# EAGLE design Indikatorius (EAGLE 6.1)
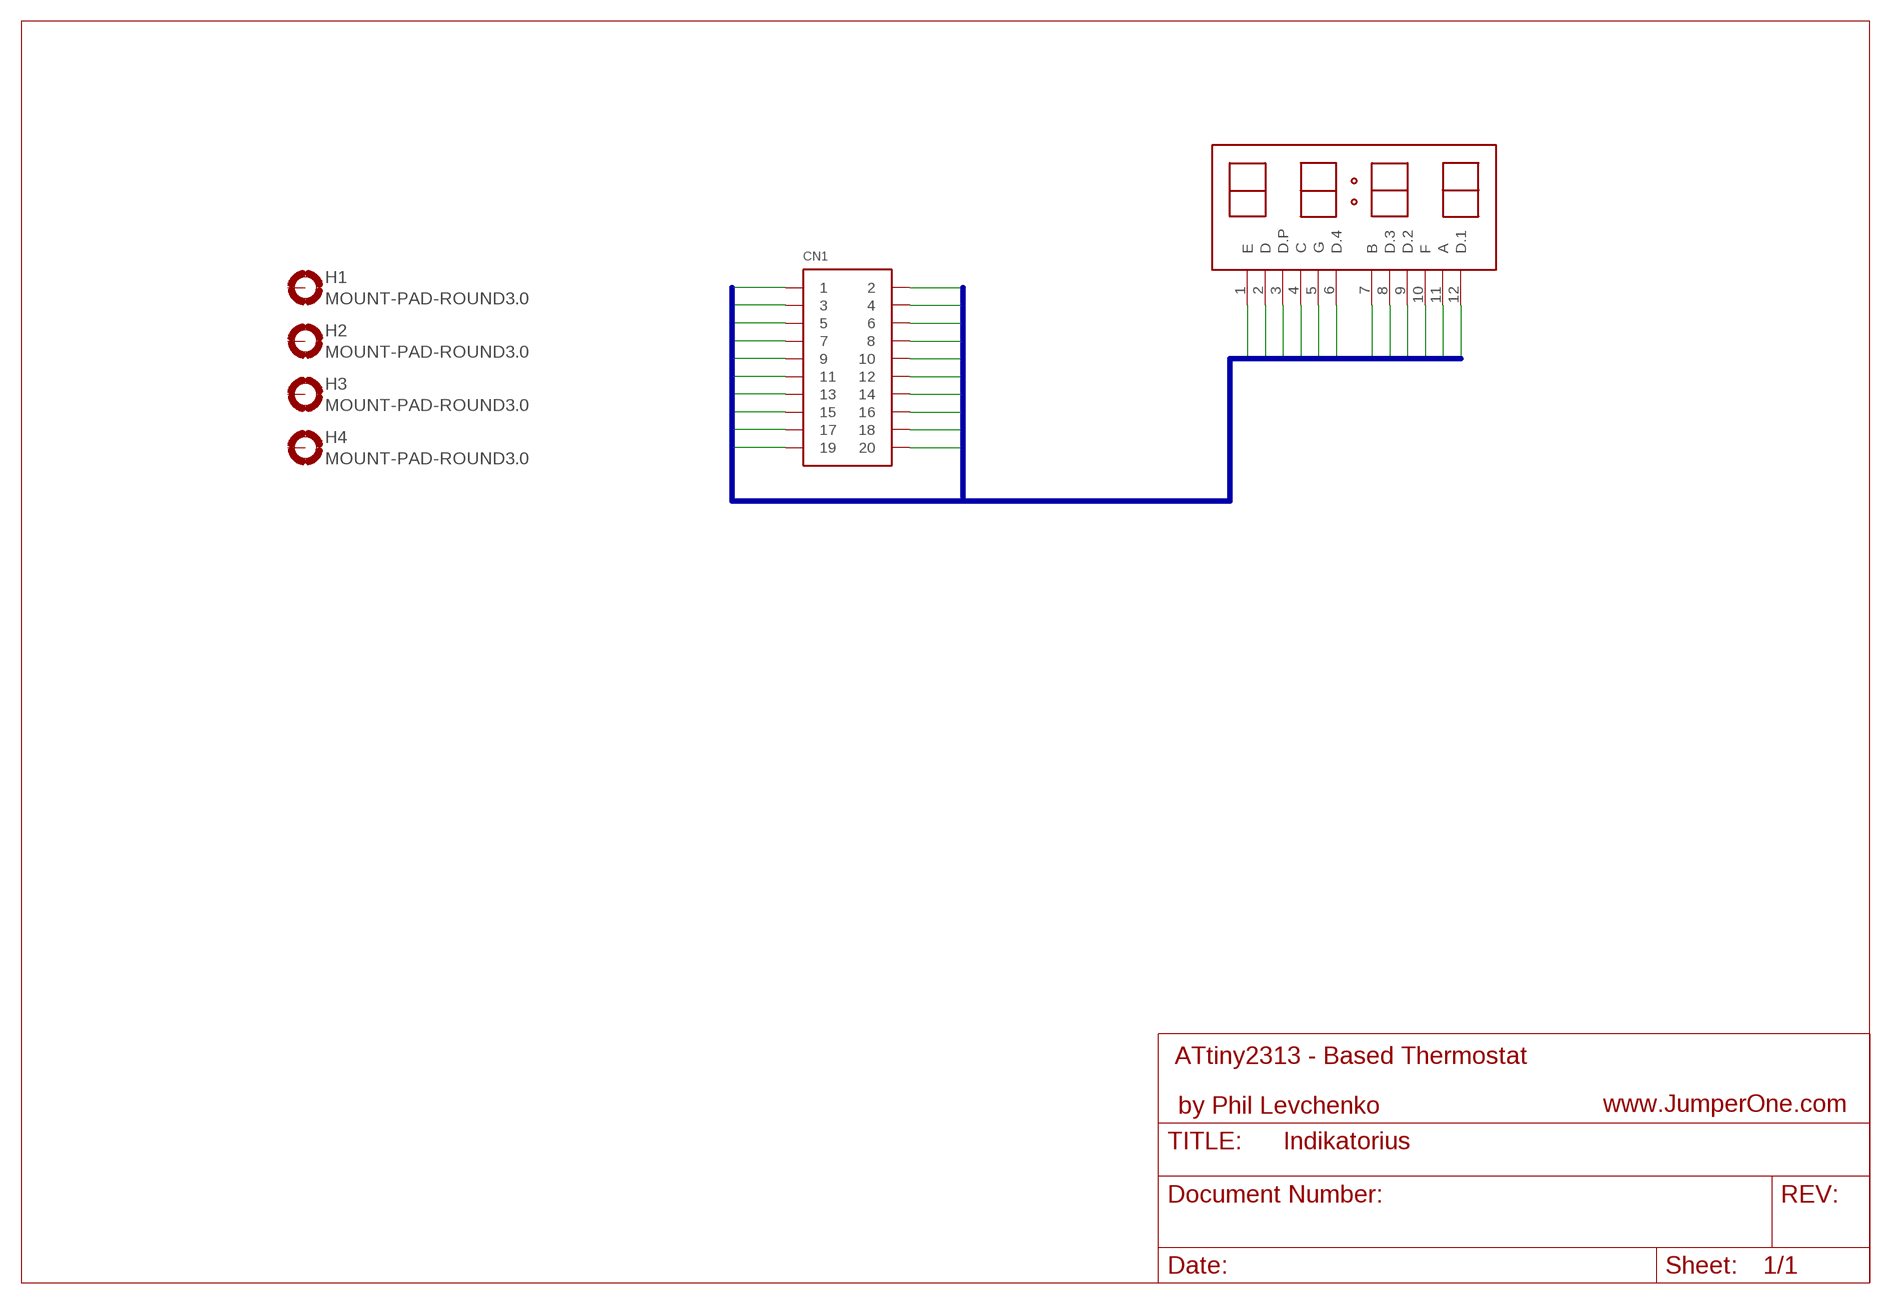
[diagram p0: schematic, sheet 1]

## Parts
CN1  CON-2X10-PH-SMD  [CON-PH-SMD-2X10]
H1  MOUNT-PAD-ROUND3.0  [3,0-PAD]
H2  MOUNT-PAD-ROUND3.0  [3,0-PAD]
H3  MOUNT-PAD-ROUND3.0  [3,0-PAD]
H4  MOUNT-PAD-ROUND3.0  [3,0-PAD]
U$1  CA56-21  [CA56-21]

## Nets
1: CN1.2 U$1.12(D.1)
2: CN1.8 U$1.9(D.2)
3: CN1.10 U$1.8(D.3)
4: CN1.11 U$1.6(D.4)
A: CN1.4 U$1.11(A)
B: CN1.12 U$1.7(B)
C: CN1.7 U$1.4(C)
D: CN1.3 U$1.2(D)
DP: CN1.5 U$1.3(D.P)
E: CN1.1 U$1.1(E)
F: CN1.6 U$1.10(F)
G: CN1.9 U$1.5(G)
GND: CN1.13 CN1.14 CN1.15 CN1.16 CN1.17 CN1.18 CN1.19 CN1.20
Unconnected: H1.B3,0(MOUNT) H2.B3,0(MOUNT) H3.B3,0(MOUNT) H4.B3,0(MOUNT)

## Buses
B$1

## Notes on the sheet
- ATtiny2313 - Based Thermostat
- by Phil Levchenko | www.JumperOne.com

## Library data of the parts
CN1 = JumperOne:CON-2X10
H1-H4 = holes:MOUNT-PAD-ROUND: MOUNTING PAD, round
U$1 = CA56-21:CA56-21

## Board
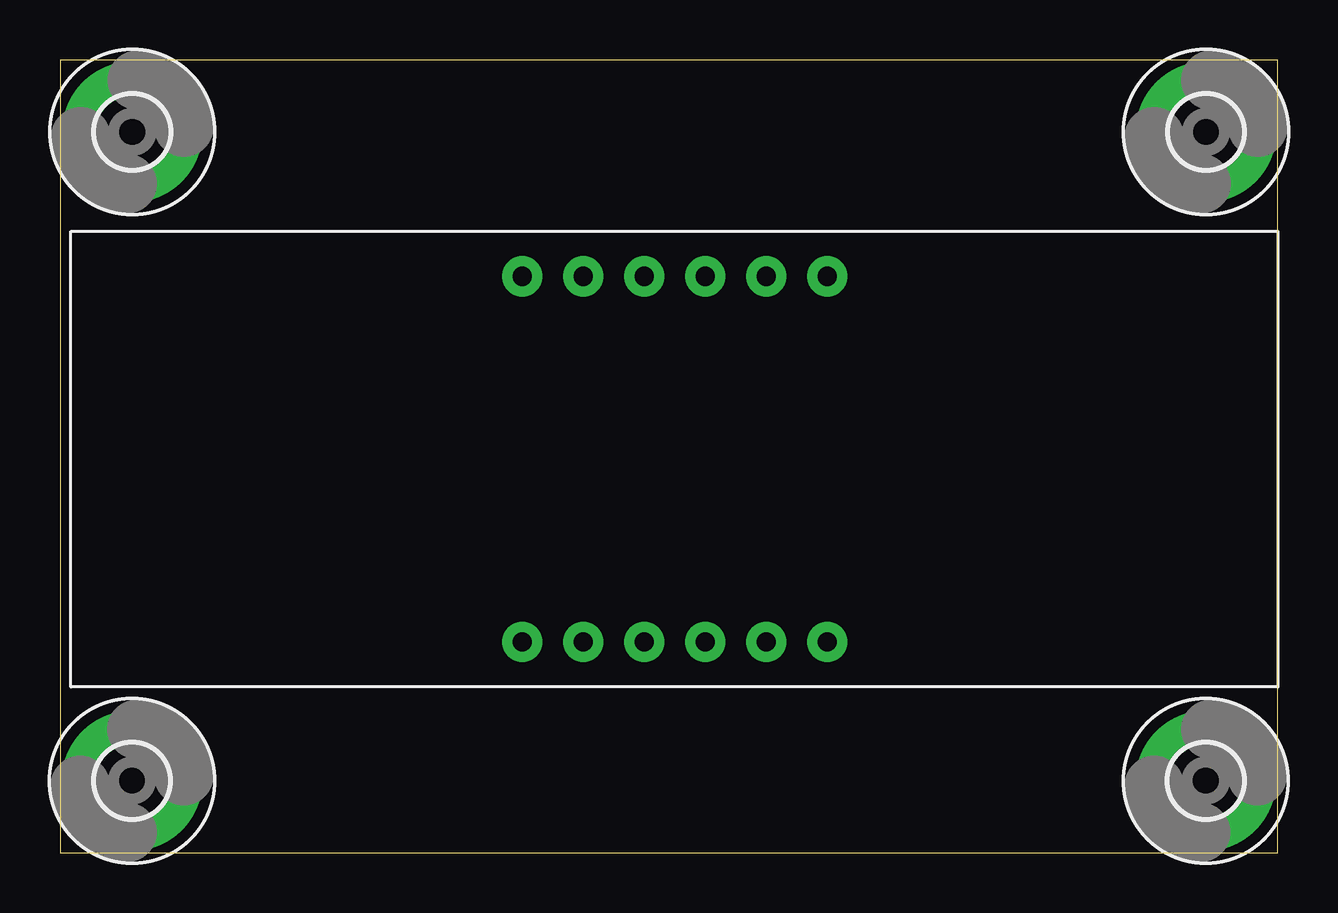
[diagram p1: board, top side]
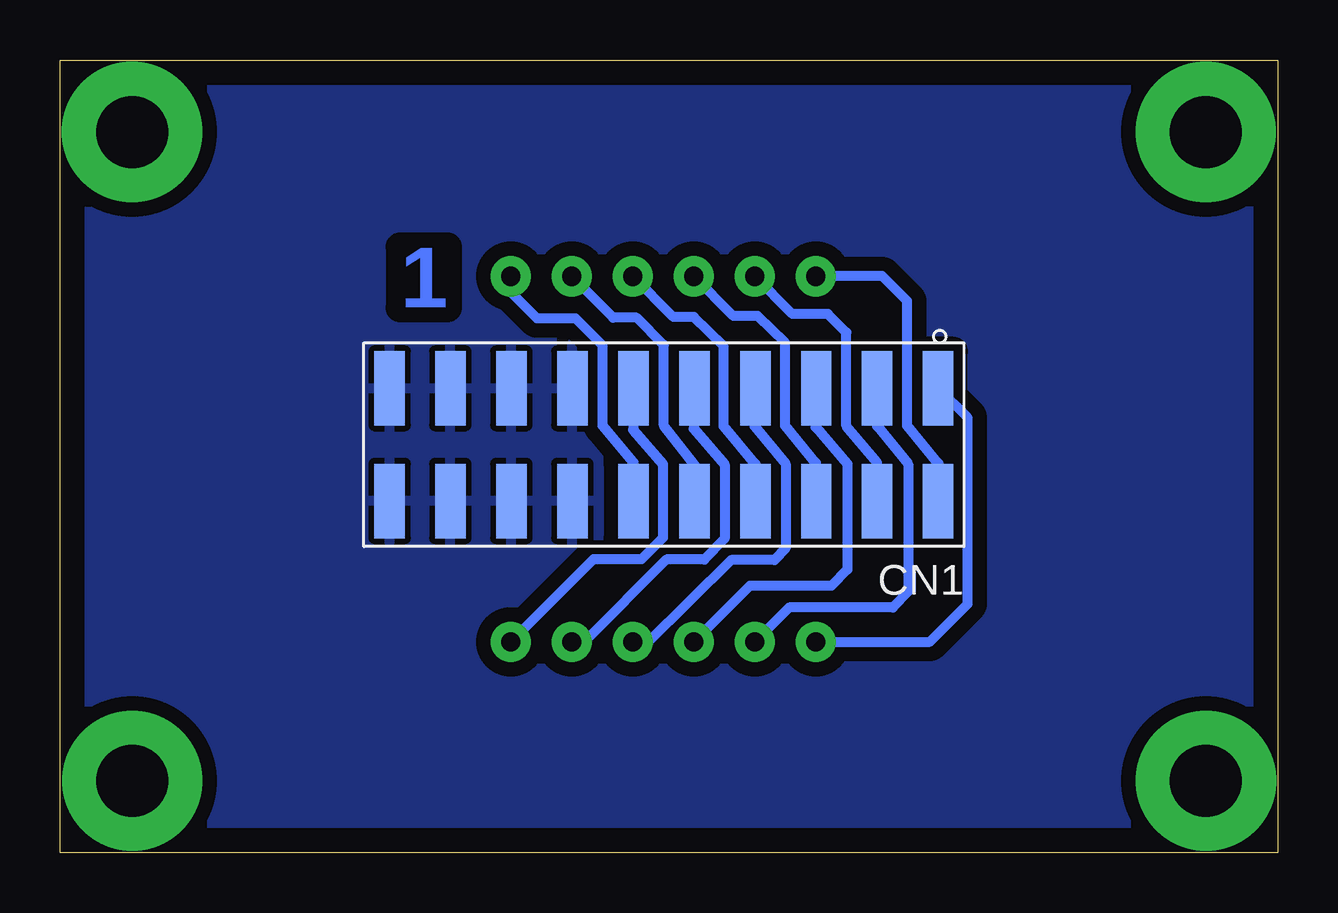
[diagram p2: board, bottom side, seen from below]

Size 50.75 x 33.05 mm. Coordinates in mm from the lower left corner, seen from the top.
Outline: 0,0 50.74,0 50.75,33.05 0.01,33.05 0,0
Copper layers (1*16): Top 0.035mm / dielectric 1.5mm / Bottom 0.035mm
Design rules: minimum track width 10mil, minimum drill 24mil, track to track 8mil, track to pad 8mil, pad to pad 8mil, via to via 8mil, smd to smd 8mil, copper to edge 40mil, drill to drill 8mil, minimum pad ring 10mil, minimum via ring 8mil, stop-mask expansion 4mil, vias tented up to drill 0mil, thermal gap 10mil

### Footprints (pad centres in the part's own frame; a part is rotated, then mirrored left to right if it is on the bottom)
CON-PH-SMD-2X10 = smd 1.27 x 3.1: 1 -11.43,-2.35; 2 -11.43,2.35; 3 -8.89,-2.35; 4 -8.89,2.35; 5 -6.35,-2.35; 6 -6.35,2.35; 7 -3.81,-2.35; 8 -3.81,2.35; 9 -1.27,-2.35; 10 -1.27,2.35; 11 1.27,-2.35; 12 1.27,2.35; 13 3.81,-2.35; 14 3.81,2.35; 15 6.35,-2.35; 16 6.35,2.35; 17 8.89,-2.35; 18 8.89,2.35; 19 11.43,-2.35; 20 11.43,2.35
3,0-PAD = drill 3 pad 5.842: B3,0 0,0
CA56-21 = drill 0.8 pad 1.676: 1 18.815,1.844; 2 21.355,1.844; 3 23.895,1.844; 4 26.435,1.844; 5 28.975,1.844; 6 31.515,1.844; 7 31.515,17.084; 8 28.975,17.084; 9 26.435,17.084; 10 23.895,17.084; 11 21.355,17.084; 12 18.815,17.084

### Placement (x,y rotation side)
CN1  25.59,17.01 180 bottom
H1  47.75,30.05 0 top
H2  3.01,30.05 0 top
H3  47.74,3 0 top
H4  3,3 0 top
U$1  0.45,6.95 0 top

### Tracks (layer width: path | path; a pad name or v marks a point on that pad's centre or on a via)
1
  Bottom 0.406: CN1.2 14.15,16.23 15.46,17.81 15.46,23 16.49,24.04 U$1.12 | 19.31,24.02 19.29,24.04 U$1.12 | U$1.12
2
  Bottom 0.406: CN1.8 21.78,16.21 23.09,17.78 23.09,21.12 24.34,22.34 25.19,22.34 U$1.9
3
  Bottom 0.406: CN1.10 24.31,16.18 25.59,17.81 25.59,21.18 26.72,22.31 27.7,22.31 U$1.8
4
  Bottom 0.406: CN1.11 26.86,17.63 25.63,16.2 25.63,13.13 26.53,12.23 28.53,12.23 U$1.6
A
  Bottom 0.406: CN1.4 16.7,16.26 17.99,17.79 17.99,21.7 18.75,22.46 20.23,22.46 U$1.11
B
  Bottom 0.406: CN1.12 26.86,16.29 28.14,17.8 28.14,21.15 29.26,22.27 30.87,22.27 32.01,23.42 32.01,23.98 U$1.7
C
  Bottom 0.406: CN1.7 21.8,17.78 20.52,16.21 20.52,12.7 20.97,12.2 22.79,12.2 26.28,8.75 26.84,8.75 U$1.4
D
  Bottom 0.406: CN1.3 16.7,17.79 15.41,16.2 15.41,10.89 16.04,10.23 20.37,10.23 U$1.2
DP
  Bottom 0.406: CN1.5 19.26,17.75 17.94,16.21 17.94,11.8 18.61,11.13 22.01,11.13 U$1.3
E
  Bottom 0.406: U$1.1 14.51,8.79 12.93,10.37 12.93,18.13 CN1.1
F
  Bottom 0.406: CN1.6 19.25,16.25 20.54,17.81 20.54,21.27 21.68,22.38 22.69,22.38 U$1.10
G
  Bottom 0.406: CN1.9 24.35,17.68 23.05,16.19 23.05,13.09 23.9,12.23 25.48,12.23 28.88,8.8 29.41,8.8 U$1.5
GND
  pour Bottom (isolate 0.6): 0.09,33.03 50.8,33.03 50.8,-0.04 0.09,-0.04

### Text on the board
Bottom: 1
